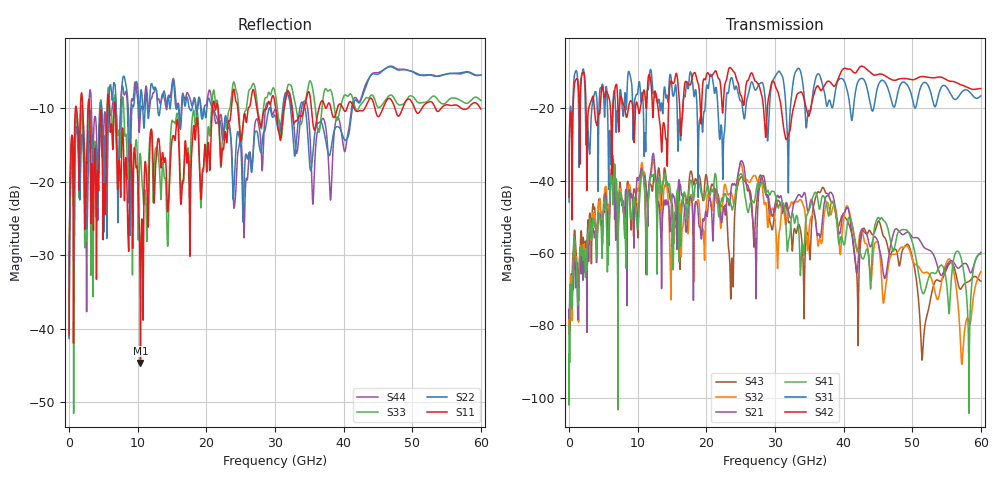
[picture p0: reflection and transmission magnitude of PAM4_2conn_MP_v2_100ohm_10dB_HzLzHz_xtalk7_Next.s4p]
! Info: Touchstone file created by Circ.  Input file=FAB50GbE_2conn_Midplane_Examax_Topo2_v2_100ohm_10dB_HzLzHz.circ
# Hz S RI R 50
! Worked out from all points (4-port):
!   6000 points, 10 MHz to 60 GHz, reference 50 ohm
!   strongest paths, dB at 10 MHz, 15.01 GHz, 30.01 GHz, 45.01 GHz, 60 GHz:
!     S42: -44.6, -12.9, -13.6, -10.6, -14.5
!     S31: -45.9, -14.7, -11.2, -13.9, -16.5
!     S41: -88.0, -53.5, -43.7, -50.2, -60.3
!     S21: -75.6, -44.1, -46.6, -57.0, -59.9
!     S32: -82.6, -53.9, -50.9, -57.0, -65.2
!     S43: -77.3, -46.7, -48.3, -51.3, -67.8
!   lowest |S11| = -44.6 dB at 10.4 GHz (marker M1), VSWR 1.01, Z = 50.6 + j0.208 ohm
!   |S11| at or under -10 dB: 2.992 GHz to 5.568 GHz (2.576 GHz wide, 60.2 % of centre); 6.762 GHz to 20.91 GHz (14.15 GHz wide, 102 % of centre); 21.7 GHz to 23.65 GHz (1.948 GHz wide, 8.59 % of centre)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
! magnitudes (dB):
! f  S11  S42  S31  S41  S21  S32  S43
! 10 MHz  -40.8  -44.6  -45.9  -88.0  -75.6  -82.6  -77.3
! 960 MHz  -9.8  -12.1  -9.7  -62.1  -69.7  -64.2  -58.0
! 10.4 GHz  -44.6  -19.6  -15.8  -41.8  -38.0  -37.8  -40.1
! 14.92 GHz  -15.0  -12.5  -12.4  -46.9  -47.2  -62.2  -45.9
! 23.67 GHz  -9.8  -9.1  -11.5  -47.4  -41.5  -43.5  -63.1
! 25.01 GHz  -14.4  -16.3  -17.9  -38.1  -34.6  -35.2  -39.1
! 60 GHz  -10.1  -14.5  -16.5  -60.3  -59.9  -65.2  -67.8
